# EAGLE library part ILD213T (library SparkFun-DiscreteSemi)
Dual Channel Phototransistor Optocoupler Dual Channel 70 V 4000 Vrms Phototransistor Optocoupler in a standard SOIC-8 package. Used to couple signals between electrically isolated circuits. Datasheet SparkFun Products: SparkFun Opto-Isolator Breakout
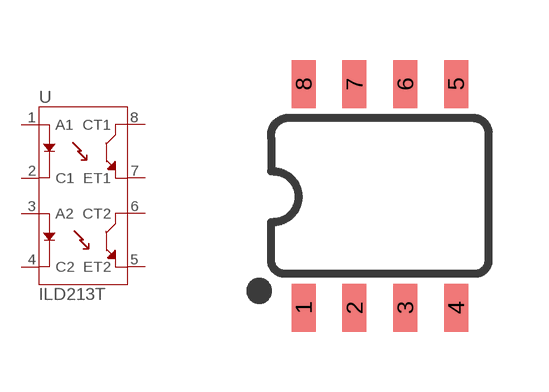
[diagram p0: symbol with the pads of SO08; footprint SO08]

Designator prefix U

## ILD213T-IDL213T (PROD_ID: IC-09076)  [SO08]
1  A1
2  C1
3  A2
4  C2
5  ET2
6  CT2
7  ET1
8  CT1

## Footprint SO08 (pad centres in mm)
SOIC, 0.15 inch width
smd 0.6 x 1.2: 1 -1.905,-2.8; 2 -0.635,-2.8; 3 0.635,-2.8; 4 1.905,-2.8; 5 1.905,2.8; 6 0.635,2.8; 7 -0.635,2.8; 8 -1.905,2.8

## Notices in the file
Licensing: Creative Commons ShareAlike 4.0 International - https://creativecommons.org/licenses/by-sa/4.0
